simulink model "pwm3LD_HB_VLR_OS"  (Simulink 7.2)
settings: Solver=ode3  SolverMode=SingleTasking  StartTime=0.0  StopTime=0.1  FixedStep=10e-6  MaxStep=1e-4  RelTol=1e-3
PreLoadFcn:
  | INIT_PWM_3L

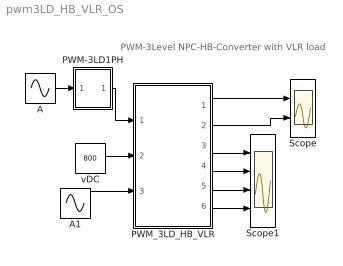
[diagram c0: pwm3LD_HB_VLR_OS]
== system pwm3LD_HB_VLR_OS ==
  note: PWM-3Level NPC-HB-Converter with VLR load
  A : Sin  Amplitude=.8  Frequency=2*pi*50  Phase=[0 ]  SampleTime=0
  A1 : Sin  Amplitude=0  Frequency=2*pi*50  Phase=[0 ]  SampleTime=0
  PWM-3LD1PH : Subsystem  mask(PWM-3LD_1PH){FT=900, PHT=0, A=0.5, O1=0.5, O2=-0.5, DT=1e-6}
      mask prompts: FT "Frequency of Trian Sig."; PHT "Phase Angle of Trian. Sig."; A "Amplitude of Trian. Sig."; O1 "Offset of 1st Trian"; O2 "Offset of 2nd Trian."; DT "Dead Time"
      mask help: Pulse Width Modulation for 1 Leg of 3 Level Neutral point clamped Converter
  PWM_3LD_HB_VLR : Subsystem  mask(pwm_3LD_HB_VLR_OS){RL=0.5, LL=2e-3}
      mask prompts: RL "Load Resistance"; LL "Load Inductance"
      mask help: Open Source 3-Level NPC PWM HB Converter with VLR load Input Vector u: u[0]= L3L1_TD1.gate u[1]= L3L1_TD2.gate u[2]= L3L1_TD3.gate u[3]= L3L1_TD4.gate u[4]= VDC u[5]= Ea Output Vector y: y[0]= Va.v, Output Voltage to middle point y[1]= Ia.I, Output AC Current y[2]= T1.I y[3]= D1.I y[4]= T1.V y[5]= T2.I y[6]= D2.I y[7]= T2.V y[8]= D5.I y[9]= D5.V y[10]= IDC1, Input DC Current y[11]= IDC2, Input DC Current Parameter Vector p: p[0]=RL p[1]=LL You can pause the simulation during running, change the Parameters you want and continue the Simulation
  Scope : Scope  NumInputPorts=2
  Scope1 : Scope  NumInputPorts=4
  vDC : Constant  Value=800  OutDataType=sfix(16)  OutScaling=2^0
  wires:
  A/1 -> PWM-3LD1PH/1(In1)
  PWM_3LD_HB_VLR/3("iT1, iD1,vT1") -> Scope1/1
  PWM_3LD_HB_VLR/4("iT2, iD2,vT2") -> Scope1/2
  PWM_3LD_HB_VLR/5(iD5,vD5) -> Scope1/3
  PWM_3LD_HB_VLR/6(iDC1,iDC2) -> Scope1/4
  PWM_3LD_HB_VLR/1(vA) -> Scope/1
  A1/1 -> PWM_3LD_HB_VLR/3(EA)
  vDC/1 -> PWM_3LD_HB_VLR/2(vDC)
  PWM-3LD1PH/1(Out1) -> PWM_3LD_HB_VLR/1(Sw)
  PWM_3LD_HB_VLR/2(iA) -> Scope/2

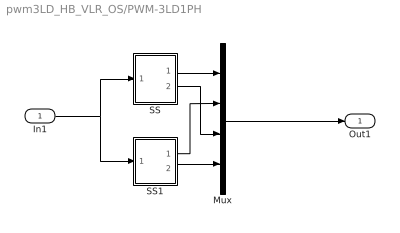
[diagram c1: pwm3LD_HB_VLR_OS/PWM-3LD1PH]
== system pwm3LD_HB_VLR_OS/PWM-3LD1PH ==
  In1 : Inport  OutDataType=sfix(16)  OutScaling=2^0
  Mux : Mux
  SS : Subsystem
  SS1 : Subsystem
  Out1 : Outport
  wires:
  SS1/2(O2) -> Mux/4
  SS/1(O1) -> Mux/1
  Mux/1 -> Out1/1
  SS/2(O2) -> Mux/3
  SS1/1(O1) -> Mux/2
  In1/1 -> SS/1(I1), SS1/1(I1)

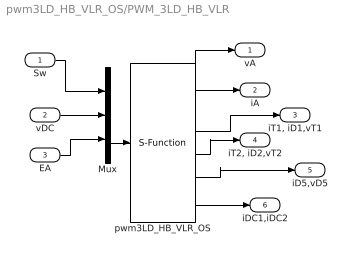
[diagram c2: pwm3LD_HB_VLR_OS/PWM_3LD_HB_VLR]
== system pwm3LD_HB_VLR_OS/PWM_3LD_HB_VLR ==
  Sw : Inport  OutDataType=sfix(16)  OutScaling=2^0
  vDC : Inport  Port=2  OutDataType=sfix(16)  OutScaling=2^0
  EA : Inport  Port=3  OutDataType=sfix(16)  OutScaling=2^0
  Mux : Mux  Inputs="[4  1 1]"
  pwm3LD_HB_VLR_OS : S-Function  FunctionName=s_pwm_3LD_HB_VLR_OS  Parameters="[RL  LL]"  EnableBusSupport=off
  vA : Outport  OutDataType=sfix(16)  OutScaling=2^0
  iA : Outport  Port=2  OutDataType=sfix(16)  OutScaling=2^0
  "iT1, iD1,vT1" : Outport  Port=3  OutDataType=sfix(16)  OutScaling=2^0
  "iT2, iD2,vT2" : Outport  Port=4  OutDataType=sfix(16)  OutScaling=2^0
  iD5,vD5 : Outport  Port=5  OutDataType=sfix(16)  OutScaling=2^0
  iDC1,iDC2 : Outport  Port=6  OutDataType=sfix(16)  OutScaling=2^0
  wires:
  pwm3LD_HB_VLR_OS/6 -> iDC1,iDC2/1
  pwm3LD_HB_VLR_OS/5 -> iD5,vD5/1
  pwm3LD_HB_VLR_OS/4 -> "iT2, iD2,vT2"/1
  pwm3LD_HB_VLR_OS/3 -> "iT1, iD1,vT1"/1
  pwm3LD_HB_VLR_OS/2 -> iA/1
  pwm3LD_HB_VLR_OS/1 -> vA/1
  EA/1 -> Mux/3
  Mux/1 -> pwm3LD_HB_VLR_OS/1
  vDC/1 -> Mux/2
  Sw/1 -> Mux/1

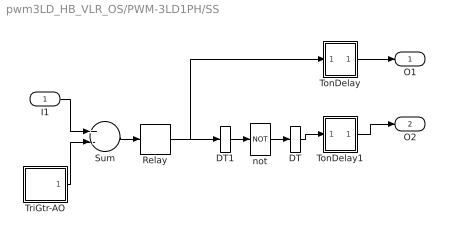
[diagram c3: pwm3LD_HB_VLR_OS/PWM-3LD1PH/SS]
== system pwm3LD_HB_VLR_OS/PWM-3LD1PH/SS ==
  I1 : Inport  OutDataType=sfix(16)  OutScaling=2^0
  DT : DataTypeConversion
  DT1 : DataTypeConversion
  Relay : Relay  OutDataType=sfix(16)  OutScaling=2^0
  Sum : Sum  Inputs=+-  OutDataType=sfix(16)  OutScaling=2^0
  TonDelay : Subsystem  mask(TonDelay){DT=DT}
      mask prompts: DT "Dead Time"
      mask help: Turn on dead time to protect against short circuit of the converter leg
  TonDelay1 : Subsystem  mask(TonDelay){DT=DT}
      mask prompts: DT "Dead Time"
      mask help: Turn on dead time to protect against short circuit of the converter leg
  TriGtr-AO : Subsystem  mask(TriGtr-AO){A=A, O=O1, T=1/FT, Td=PHT/FT/180}
      mask prompts: A "Amplitude"; O "Offset"; T "Period Time"; Td "Time Delay"
      mask help: Triangular Wave Generator with variable time delay, variable amplitude and offset
  not : Logic  Operator=NOT  Inputs=1
  O1 : Outport  InitialOutput=0
  O2 : Outport  Port=2  InitialOutput=0
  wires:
  DT1/1 -> not/1
  DT/1 -> TonDelay1/1(s1)
  I1/1 -> Sum/1
  TriGtr-AO/1(Out1) -> Sum/2
  Sum/1 -> Relay/1
  not/1 -> DT/1
  TonDelay1/1(s1d) -> O2/1
  Relay/1 -> DT1/1, TonDelay/1(s1)
  TonDelay/1(s1d) -> O1/1

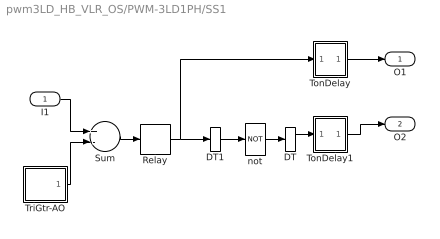
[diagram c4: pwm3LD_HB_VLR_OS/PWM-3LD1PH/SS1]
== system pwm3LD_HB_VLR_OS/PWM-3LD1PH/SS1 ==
  I1 : Inport  OutDataType=sfix(16)  OutScaling=2^0
  DT : DataTypeConversion
  DT1 : DataTypeConversion
  Relay : Relay  OutDataType=sfix(16)  OutScaling=2^0
  Sum : Sum  Inputs=+-  OutDataType=sfix(16)  OutScaling=2^0
  TonDelay : Subsystem  mask(TonDelay){DT=DT}
      mask prompts: DT "Dead Time"
      mask help: Turn on dead time to protect against short circuit of the converter leg
  TonDelay1 : Subsystem  mask(TonDelay){DT=DT}
      mask prompts: DT "Dead Time"
      mask help: Turn on dead time to protect against short circuit of the converter leg
  TriGtr-AO : Subsystem  mask(TriGtr-AO){A=A, O=O2, T=1/FT, Td=PHT/FT/180}
      mask prompts: A "Amplitude"; O "Offset"; T "Period Time"; Td "Time Delay"
      mask help: Triangular Wave Generator with variable time delay, variable amplitude and offset
  not : Logic  Operator=NOT  Inputs=1
  O1 : Outport  InitialOutput=0
  O2 : Outport  Port=2  InitialOutput=0
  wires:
  DT1/1 -> not/1
  DT/1 -> TonDelay1/1(s1)
  I1/1 -> Sum/1
  TriGtr-AO/1(Out1) -> Sum/2
  Sum/1 -> Relay/1
  not/1 -> DT/1
  TonDelay1/1(s1d) -> O2/1
  Relay/1 -> DT1/1, TonDelay/1(s1)
  TonDelay/1(s1d) -> O1/1

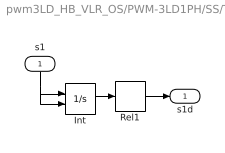
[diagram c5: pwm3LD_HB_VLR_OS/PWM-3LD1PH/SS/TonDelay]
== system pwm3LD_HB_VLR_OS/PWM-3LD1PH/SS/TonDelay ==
  s1 : Inport  Orientation=down  OutDataType=sfix(16)  OutScaling=2^0
  Int : Integrator  ExternalReset=falling
  Rel1 : Relay  OnSwitchValue=DT  OutDataType=sfix(16)  OutScaling=2^0
  s1d : Outport  InitialOutput=0
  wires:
  Int/1 -> Rel1/1
  s1/1 -> Int/2, Int/1
  Rel1/1 -> s1d/1

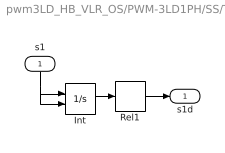
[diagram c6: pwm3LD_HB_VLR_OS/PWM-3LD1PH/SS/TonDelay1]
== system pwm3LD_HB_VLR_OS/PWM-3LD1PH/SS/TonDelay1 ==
  s1 : Inport  Orientation=down  OutDataType=sfix(16)  OutScaling=2^0
  Int : Integrator  ExternalReset=falling
  Rel1 : Relay  OnSwitchValue=DT  OutDataType=sfix(16)  OutScaling=2^0
  s1d : Outport  InitialOutput=0
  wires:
  Int/1 -> Rel1/1
  s1/1 -> Int/2, Int/1
  Rel1/1 -> s1d/1

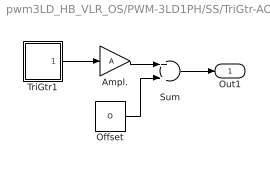
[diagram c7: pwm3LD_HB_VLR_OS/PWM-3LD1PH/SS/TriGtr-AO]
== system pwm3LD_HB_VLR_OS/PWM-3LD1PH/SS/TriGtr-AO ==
  Ampl. : Gain  Gain=A  ParameterDataType=sfix(16)  ParameterScaling=2^0  OutDataType=sfix(16)  OutScaling=2^0
  Offset : Constant  Value=O  OutDataType=sfix(16)  OutScaling=2^0
  Sum : Sum  OutDataType=sfix(16)  OutScaling=2^0
  TriGtr1 : Subsystem  mask(TriGtr){T=T, Td=Td}
      mask prompts: T "Period Time"; Td "Time Delay"
      mask help: Triangular Wave Generator with variable time delay
  Out1 : Outport
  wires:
  Offset/1 -> Sum/2
  TriGtr1/1(O) -> Ampl./1
  Ampl./1 -> Sum/1
  Sum/1 -> Out1/1

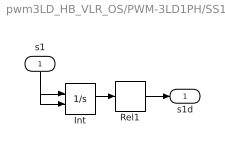
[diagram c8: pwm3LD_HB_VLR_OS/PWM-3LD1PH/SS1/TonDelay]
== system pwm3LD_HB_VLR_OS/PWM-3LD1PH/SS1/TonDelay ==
  s1 : Inport  Orientation=down  OutDataType=sfix(16)  OutScaling=2^0
  Int : Integrator  ExternalReset=falling
  Rel1 : Relay  OnSwitchValue=DT  OutDataType=sfix(16)  OutScaling=2^0
  s1d : Outport  InitialOutput=0
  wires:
  Int/1 -> Rel1/1
  s1/1 -> Int/2, Int/1
  Rel1/1 -> s1d/1

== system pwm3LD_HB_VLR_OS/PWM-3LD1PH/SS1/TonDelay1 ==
  s1 : Inport  Orientation=down  OutDataType=sfix(16)  OutScaling=2^0
  Int : Integrator  ExternalReset=falling
  Rel1 : Relay  OnSwitchValue=DT  OutDataType=sfix(16)  OutScaling=2^0
  s1d : Outport  InitialOutput=0
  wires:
  Int/1 -> Rel1/1
  s1/1 -> Int/2, Int/1
  Rel1/1 -> s1d/1

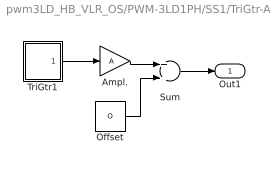
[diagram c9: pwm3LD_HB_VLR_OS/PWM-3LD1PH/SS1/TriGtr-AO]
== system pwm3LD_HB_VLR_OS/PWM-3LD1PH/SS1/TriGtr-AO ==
  Ampl. : Gain  Gain=A  ParameterDataType=sfix(16)  ParameterScaling=2^0  OutDataType=sfix(16)  OutScaling=2^0
  Offset : Constant  Value=O  OutDataType=sfix(16)  OutScaling=2^0
  Sum : Sum  OutDataType=sfix(16)  OutScaling=2^0
  TriGtr1 : Subsystem  mask(TriGtr){T=T, Td=Td}
      mask prompts: T "Period Time"; Td "Time Delay"
      mask help: Triangular Wave Generator with variable time delay
  Out1 : Outport
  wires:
  Sum/1 -> Out1/1
  Ampl./1 -> Sum/1
  TriGtr1/1(O) -> Ampl./1
  Offset/1 -> Sum/2

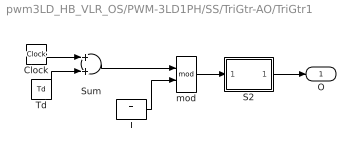
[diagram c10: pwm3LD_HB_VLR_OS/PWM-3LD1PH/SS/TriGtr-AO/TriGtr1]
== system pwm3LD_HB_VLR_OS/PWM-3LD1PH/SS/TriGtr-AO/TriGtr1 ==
  Clock : Clock
  S2 : Subsystem
  Sum : Sum  OutDataType=sfix(16)  OutScaling=2^0
  T : Constant  Value=T  OutDataType=sfix(16)  OutScaling=2^0
  Td : Constant  Value=Td  OutDataType=sfix(16)  OutScaling=2^0
  mod : Math  Operator=mod
  O : Outport  InitialOutput=0
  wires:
  mod/1 -> S2/1(I1)
  S2/1(O1) -> O/1
  Clock/1 -> Sum/1
  T/1 -> mod/2
  Sum/1 -> mod/1
  Td/1 -> Sum/2

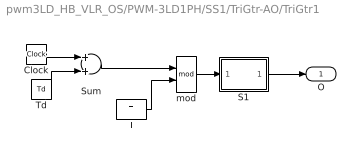
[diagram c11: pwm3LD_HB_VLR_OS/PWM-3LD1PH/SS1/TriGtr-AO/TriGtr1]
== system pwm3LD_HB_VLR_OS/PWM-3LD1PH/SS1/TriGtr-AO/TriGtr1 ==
  Clock : Clock
  S1 : Subsystem
  Sum : Sum
  T : Constant  Value=T
  Td : Constant  Value=Td
  mod : Math  Operator=mod
  O : Outport  InitialOutput=0
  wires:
  mod/1 -> S1/1(I1)
  S1/1(O1) -> O/1
  Clock/1 -> Sum/1
  T/1 -> mod/2
  Sum/1 -> mod/1
  Td/1 -> Sum/2

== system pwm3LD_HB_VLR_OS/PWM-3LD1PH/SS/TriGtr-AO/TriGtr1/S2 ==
  I1 : Inport
  Fcn : Fcn  Expr="(u* (u <=T/4) * 4/T)   +  (  (u > T/4) && ( u <=3*T/4) )* ( 1 - (u-T/4) *4/T )   +  ( (u > 3*T/4)&& (u<=T)) * ( ((u -3*T/4)* 4/T )-1 )"
  O1 : Outport
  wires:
  I1/1 -> Fcn/1
  Fcn/1 -> O1/1

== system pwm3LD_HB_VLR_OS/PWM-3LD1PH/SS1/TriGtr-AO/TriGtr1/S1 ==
  I1 : Inport
  Fcn : Fcn  Expr="(u* (u <=T/4) * 4/T)   +  (  (u > T/4) && ( u <=3*T/4) )* ( 1 - (u-T/4) *4/T )   +  ( (u > 3*T/4)&& (u<=T)) * ( ((u -3*T/4)* 4/T )-1 )"
  O1 : Outport
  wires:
  Fcn/1 -> O1/1
  I1/1 -> Fcn/1
